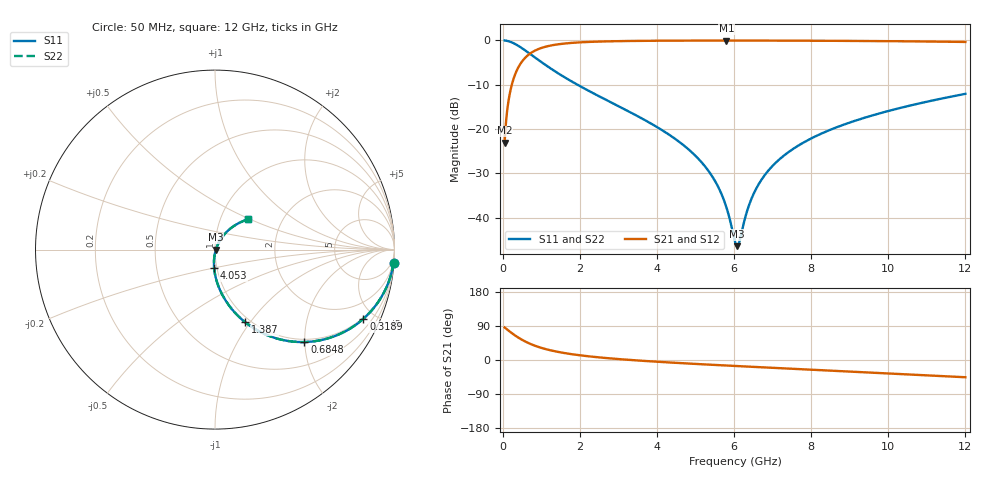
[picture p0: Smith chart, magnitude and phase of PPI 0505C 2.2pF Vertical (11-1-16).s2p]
# GHz S MA R 50
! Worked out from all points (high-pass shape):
!   1601 points, 50 MHz to 12 GHz, reference 50 ohm
!   highest |S21| = -0.04 dB at 5.801 GHz (marker M1); lowest = -23.1 dB at 50 MHz (marker M2)
!   |S21| within 3 dB of the highest: 699.8 MHz to end of sweep
!   lowest |S11| = -46.4 dB at 6.085 GHz (marker M3), VSWR 1.01, Z = 50.5 - j0.127 ohm
!   |S11| at or under -10 dB: 1.938 GHz to end of sweep
!   |S22| runs from -46.4 to 0.0 dB; largest |S21 - S12| = 0
!   S11 on the Smith chart (normalised r, x): 50 MHz: 1, -28; 318.9 MHz: 0.94, -4.31; 684.8 MHz: 0.94, -1.99; 1.387 GHz: 0.94, -0.95; 4.053 GHz: 0.97, -0.20; 12 GHz: 1.35, +0.49
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0.05  0.9975 -4.1  0.07003 85.8  0.07003 85.8  0.9975 -4.1
0.1769688  0.9704 -14.4  0.2413 75.6  0.2413 75.6  0.9704 -14.4
0.318875  0.9121 -25.0  0.4093 65.0  0.4093 65.0  0.9121 -25.0
0.4906563  0.8216 -36.0  0.5692 53.9  0.5692 53.9  0.8216 -36.0
0.6848437  0.7163 -46.0  0.6965 43.9  0.6965 43.9  0.7163 -46.0
1.006  0.5676 -57.9  0.8215 31.9  0.8215 31.9  0.5676 -57.9
1.386906  0.4391 -67.4  0.8963 22.4  0.8963 22.4  0.4391 -67.4
2.044156  0.2981 -77.6  0.9518 11.9  0.9518 11.9  0.2981 -77.6
4.038312  0.1029 -92.7  0.9907 -4.8  0.9907 -4.8  0.1029 -92.7
4.05325  0.102 -92.8  0.9907 -4.9  0.9907 -4.9  0.102 -92.8
5.1885  0.04069 -95.3  0.9945 -11.4  0.9945 -11.4  0.04069 -95.3
5.547  0.02411 -92.5  0.9949 -13.3  0.9949 -13.3  0.02411 -92.5
5.800937  0.01314 -84.0  0.9949 -14.6  0.9949 -14.6  0.01314 -84.0
6.025  0.005364 -43.7  0.9949 -15.7  0.9949 -15.7  0.005364 -43.7
6.08475  0.004769 -15.3  0.9948 -16.0  0.9948 -16.0  0.004769 -15.3
6.1445  0.005464 12.2  0.9948 -16.3  0.9948 -16.3  0.005464 12.2
6.428312  0.0154 53.5  0.9945 -17.8  0.9945 -17.8  0.0154 53.5
6.749469  0.02831 60.3  0.9941 -19.4  0.9941 -19.4  0.02831 60.3
7.272281  0.04929 61.8  0.993 -21.9  0.993 -21.9  0.04929 61.8
8.019156  0.07899 60.3  0.9906 -25.5  0.9906 -25.5  0.07899 60.3
10.01331  0.1602 52.2  0.9796 -35.3  0.9796 -35.3  0.1602 52.2
12  0.2494 42.6  0.9594 -45.5  0.9594 -45.5  0.2494 42.6
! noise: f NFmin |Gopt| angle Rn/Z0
0.05  0.0007281  0.9422  2.022  0.002818
1.372  0.005669  0.7601  4.729  0.004781
2.701  0.009247  0.7169  7.866  0.006428
4.031  0.01247  0.6916  11.09  0.007802
5.36  0.01555  0.6751  14.3  0.009092
6.682  0.01859  0.6644  17.47  0.01038
8.012  0.02171  0.6581  20.61  0.01175
9.341  0.02497  0.6555  23.7  0.01326
10.67  0.02843  0.6561  26.75  0.01495
12  0.03218  0.6596  29.76  0.01692
